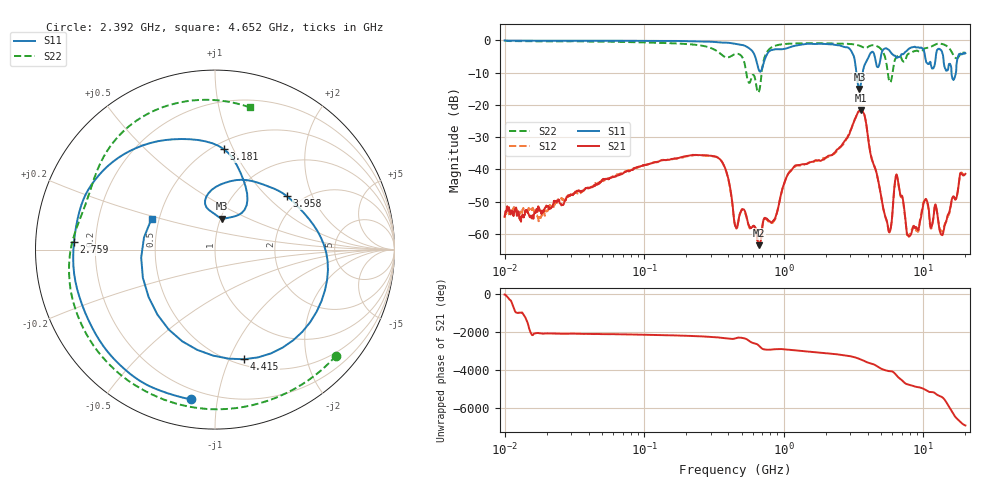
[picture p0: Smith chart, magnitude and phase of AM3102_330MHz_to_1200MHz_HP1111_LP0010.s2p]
! Date/Time: Tue, Sep 11, 2018 5:24 PM
! Network Analyzer: Agilent Technologies E8362B Rev: A.07.50.63
! Sweep from 0.010 to 20.000 GHz, 1601 Points, Sweep Type: LOG
! Power Supply: 4.949 V, 0.001 A
# Hz S DB R 50
!freq MagS11 AngS11 MagS21 AngS21 MagS12 AngS12 MagS22 AngS22
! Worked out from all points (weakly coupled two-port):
!   1601 points, 10 MHz to 20 GHz, reference 50 ohm
!   highest |S21| = -21.61 dB at 3.549 GHz (marker M1); lowest = -63.5 dB at 660.2 MHz (marker M2)
!   lowest |S11| = -15.1 dB at 3.482 GHz (marker M3), VSWR 1.43, Z = 50.5 + j18 ohm
!   |S11| at or under -10 dB: 3.313 GHz to 3.668 GHz (355.7 MHz wide, 10.2 % of centre); 15.91 GHz to 17.11 GHz (1.203 GHz wide, 7.28 % of centre)
!   |S22| runs from -16.1 to -0.1 dB; largest |S21 - S12| = 0.005
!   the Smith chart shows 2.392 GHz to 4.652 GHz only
!   S11 on the Smith chart (normalised r, x): 2.392 GHz: 0.14, -0.84; 2.759 GHz: 0.12, +0.03; 3.181 GHz: 0.57, +0.92; 3.958 GHz: 1.67, +1.33; 4.415 GHz: 0.56, -1.14; 4.652 GHz: 0.45, +0.18
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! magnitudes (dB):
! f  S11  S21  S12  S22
! 10 MHz  0.0  -54.6  -55.0  -0.1
! 35.55 MHz  -0.1  -46.9  -47.0  -0.3
! 126.4 MHz  -0.2  -37.5  -37.7  -0.7
! 341.1 MHz  -0.6  -36.5  -36.4  -3.7
! 447.2 MHz  -1.0  -57.2  -57.3  -4.2
! 660.2 MHz  -8.9  -63.5  -63.8  -16.1
! 798.4 MHz  -3.1  -56.3  -56.3  -2.5
! 1.59 GHz  -1.1  -37.7  -37.6  -0.9
! 2.392 GHz  -1.5  -33.9  -34.4  -0.9
! 2.759 GHz  -2.1  -31.0  -31.3  -1.0
! 3.181 GHz  -5.0  -25.1  -25.1  -1.2
! 3.482 GHz  -15.1  -21.9  -21.8  -1.6
! 3.549 GHz  -13.9  -21.6  -21.5  -1.7
! 3.958 GHz  -6.0  -28.1  -28.0  -2.2
! 4.415 GHz  -4.0  -38.6  -38.5  -1.5
! 4.652 GHz  -8.1  -41.6  -41.7  -1.8
! 5.652 GHz  -2.9  -59.3  -59.2  -12.1
! 6.426 GHz  -5.3  -41.5  -41.9  -5.1
! 7.845 GHz  -2.7  -60.7  -60.5  -4.1
! 10.38 GHz  -5.9  -49.2  -49.4  -2.4
! 13.55 GHz  -3.3  -60.3  -59.2  -1.1
! 20 GHz  -4.0  -41.4  -41.8  -3.8
